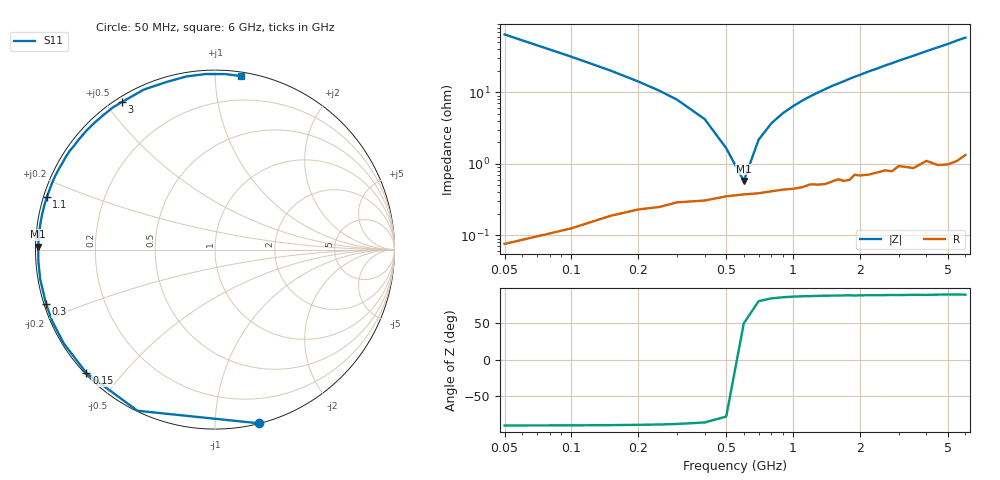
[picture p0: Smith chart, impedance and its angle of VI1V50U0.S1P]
! Infineon Technologies  Discrete & RF Semiconductors
! BB 804
! Si Tuning Diode in SOT23
! VR = 1.5 V
! S-Parameters:  July  1999
# GHz  S  MA  R  50
!  f  S11
! GHz  MAG  ANG
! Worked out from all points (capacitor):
!   34 points, 50 MHz to 6 GHz, reference 50 ohm
!   read as one part to ground: C = 49.1 pF near 50 MHz
!   lowest |Z| = 574 mohm at 600 MHz (marker M1)
!   series resonance near 578.7 MHz, so ESL is about 1.5 nH
!   S11 on the Smith chart (normalised r, x): 50 MHz: 0.00, -1.29; 150 MHz: 0.00, -0.40; 300 MHz: 0.01, -0.16; 1.1 GHz: 0.01, +0.15; 3 GHz: 0.02, +0.55; 6 GHz: 0.03, +1.16
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0.05  0.9989 -75.7
0.1  0.9964 -115.7
0.15  0.9936 -136.1
0.2  0.9915 -148.3
0.25  0.9905 -156.3
0.3  0.9888 -162.1
0.4  0.9879 -170.4
0.5  0.9861 -176.3
0.6  0.9852 179.0
0.7  0.9847 175.1
0.8  0.9837 171.6
0.9  0.9829 168.4
1.1  0.9818 162.7
1.4  0.9803 155.0
1.6  0.9776 150.3
1.7  0.9789 148.1
1.9  0.975 143.5
2.2  0.9758 137.2
2.4  0.9748 133.5
2.6  0.9739 129.4
2.8  0.9753 125.9
3  0.9719 122.2
3.5  0.9758 114.0
4  0.9723 106.2
4.5  0.9779 99.3
5  0.9796 93.1
5.5  0.9795 86.6
6  0.9776 81.5
